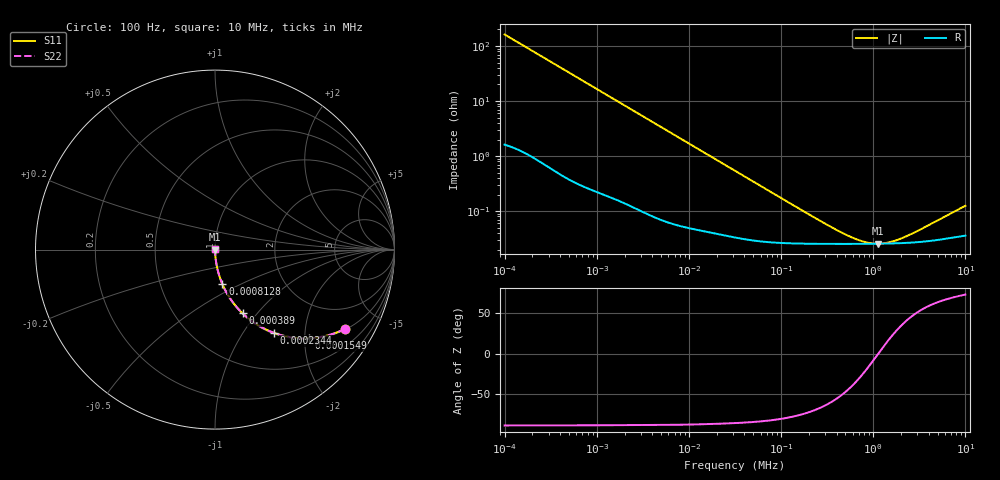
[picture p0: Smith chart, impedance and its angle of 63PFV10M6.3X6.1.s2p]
!Components F PZ-CAP
!CONCATENATE F 0.1-10000kHz, at 20deg DC=0V
!Part Number F 63PFV10M6.3X6.1
!Copyright(C) Rubycon Corporation. 20160711
# MHz S MA R 50
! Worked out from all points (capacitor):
!   501 points, 100 Hz to 10 MHz, reference 50 ohm
!   read as one part in series: C = 9.79 uF near 104.7 Hz
!   lowest |Z| = 25.5 mohm at 1.122 MHz (marker M1)
!   series resonance near 1.137 MHz, so ESL is about 2 nH
!   S11 on the Smith chart (normalised r, x): 100 Hz: 1.03, -3.24; 154.9 Hz: 1.02, -2.10; 234.4 Hz: 1.02, -1.40; 389 Hz: 1.01, -0.84; 812.8 Hz: 1.01, -0.41; 10 MHz: 1.00, +0.00
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0.0001  0.8475 -31.5  0.5224 57.9  0.5224 57.9  0.8475 -31.5
0.0001548817  0.7206 -43.2  0.6851 46.1  0.6851 46.1  0.7206 -43.2
0.0001905461  0.6468 -49.0  0.7551 40.3  0.7551 40.3  0.6468 -49.0
0.0002344229  0.569 -54.7  0.8157 34.7  0.8157 34.7  0.569 -54.7
0.0003019952  0.4746 -61.0  0.8748 28.3  0.8748 28.3  0.4746 -61.0
0.0003890451  0.3871 -66.6  0.9177 22.8  0.9177 22.8  0.3871 -66.6
0.0005128614  0.3042 -71.6  0.9491 17.7  0.9491 17.7  0.3042 -71.6
0.000691831  0.2309 -76.0  0.9702 13.3  0.9702 13.3  0.2309 -76.0
0.0008128305  0.1982 -77.8  0.9777 11.4  0.9777 11.4  0.1982 -77.8
0.001174898  0.139 -81.2  0.9883 8.0  0.9883 8.0  0.139 -81.2
0.001778279  0.09274 -83.8  0.9942 5.3  0.9942 5.3  0.09274 -83.8
0.004677351  0.03574 -86.8  0.9986 2.0  0.9986 2.0  0.03574 -86.8
0.03162278  0.005402 -86.2  0.9997 0.3  0.9997 0.3  0.005402 -86.2
0.2187762  0.0008 -71.4  0.9997 0.0  0.9997 0.0  0.0008 -71.4
0.3981072  0.0004562 -56.3  0.9997 0.0  0.9997 0.0  0.0004562 -56.3
0.6025596  0.000326 -39.1  0.9997 0.0  0.9997 0.0  0.000326 -39.1
0.8317638  0.0002712 -20.8  0.9997 0.0  0.9997 0.0  0.0002712 -20.8
1.122018  0.000255 -0.9  0.9997 0.0  0.9997 0.0  0.000255 -0.9
1.479108  0.0002694 17.4  0.9997 -0.0  0.9997 -0.0  0.0002694 17.4
1.905461  0.000307 32.0  0.9997 -0.0  0.9997 -0.0  0.000307 32.0
2.570396  0.0003813 45.6  0.9997 -0.0  0.9997 -0.0  0.0003813 45.6
10  0.00125 73.3  0.9996 -0.1  0.9996 -0.1  0.00125 73.3
